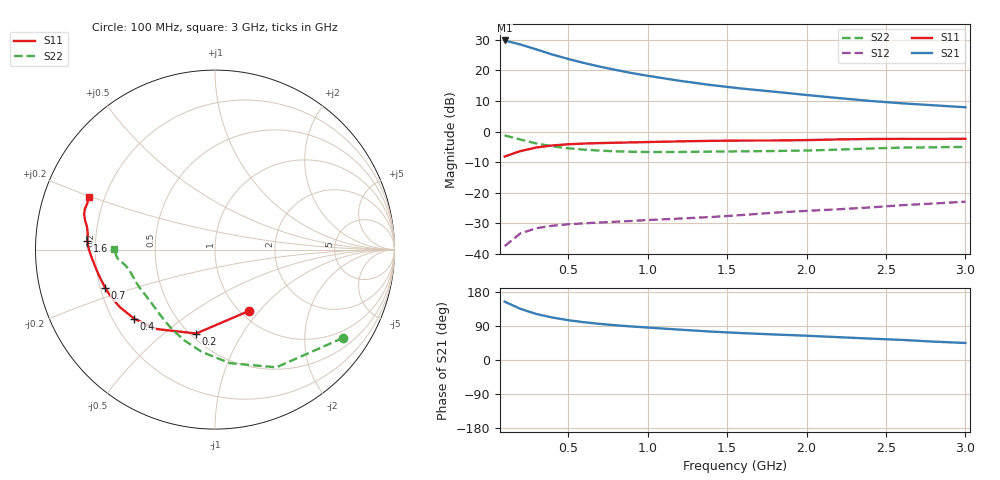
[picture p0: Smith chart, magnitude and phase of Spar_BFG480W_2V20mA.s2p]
! Filename: 220BFG480.001
! Title: BFG480W
! Bias: Vce=2V; Ic=20mA
! Company: NXP Semiconductors NL
! User: Quality&Reliability T&D
! Measure time: 10 Nov 1999 / 11:53:27
#  MHz  S  MA  R 50
! Freq  S11  S21  S12  S22  :
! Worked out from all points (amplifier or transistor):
!   20 points, 100 MHz to 3 GHz, reference 50 ohm
!   highest |S21| = 29.8 dB at 100 MHz (marker M1)
!   |S21| within 3 dB of that: start of sweep to 304.6 MHz
!   unconditionally stable (mu >= 1): 1.398 GHz to end of sweep
!   at 400 MHz: K = 0.38, MSG = 28.0 dB, |S12| = -30.8 dB
!   at 1.2 GHz: K = 0.92, MSG = 22.6 dB, |S12| = -28.5 dB
!   at 3 GHz: K = 1.17, MAG = 13.0 dB, |S12| = -23.0 dB
!   S11 on the Smith chart (normalised r, x): 100 MHz: 1.10, -0.88; 200 MHz: 0.54, -0.65; 400 MHz: 0.29, -0.34; 700 MHz: 0.22, -0.16; 1.6 GHz: 0.17, +0.03; 3 GHz: 0.14, +0.20
100  0.3907 -60.7  30.98 154.0  0.01331 68.1  0.8664 -34.6
200  0.4791 -102.6  26.57 134.9  0.02162 53.4  0.7396 -62.5
300  0.5491 -126.3  22.13 121.4  0.0262 45.2  0.6382 -82.5
400  0.5923 -139.5  18.24 112.1  0.02876 40.7  0.5745 -97.4
500  0.62 -149.0  15.44 105.1  0.03034 38.7  0.5332 -108.8
600  0.6365 -155.7  13.24 99.6  0.03148 37.9  0.5061 -117.5
700  0.6478 -160.8  11.55 95.3  0.0325 38.1  0.4877 -124.5
800  0.6565 -165.0  10.19 91.6  0.03345 39.0  0.4748 -130.2
900  0.6647 -168.4  9.071 88.5  0.03441 40.4  0.4667 -135.2
1000  0.6735 -171.7  8.187 85.6  0.0356 41.8  0.4626 -139.7
1200  0.6907 -176.8  6.788 80.2  0.03768 44.7  0.4633 -147.1
1400  0.7049 179.4  5.766 75.0  0.03992 47.6  0.4699 -152.7
1600  0.7128 176.1  5.032 70.9  0.04314 50.9  0.4751 -157.0
1800  0.7146 172.8  4.484 67.3  0.04707 53.9  0.4804 -161.3
2000  0.7248 169.8  3.967 64.1  0.05034 56.7  0.4893 -165.9
2200  0.7436 167.0  3.538 60.3  0.05344 58.6  0.5066 -170.0
2400  0.7558 164.7  3.172 56.4  0.05728 59.9  0.5289 -172.9
2600  0.7594 162.7  2.901 53.0  0.06234 61.0  0.5454 -174.9
2800  0.7568 160.1  2.692 48.5  0.06642 61.0  0.5532 -177.2
3000  0.7618 157.3  2.498 44.9  0.07119 61.5  0.5606 179.7
